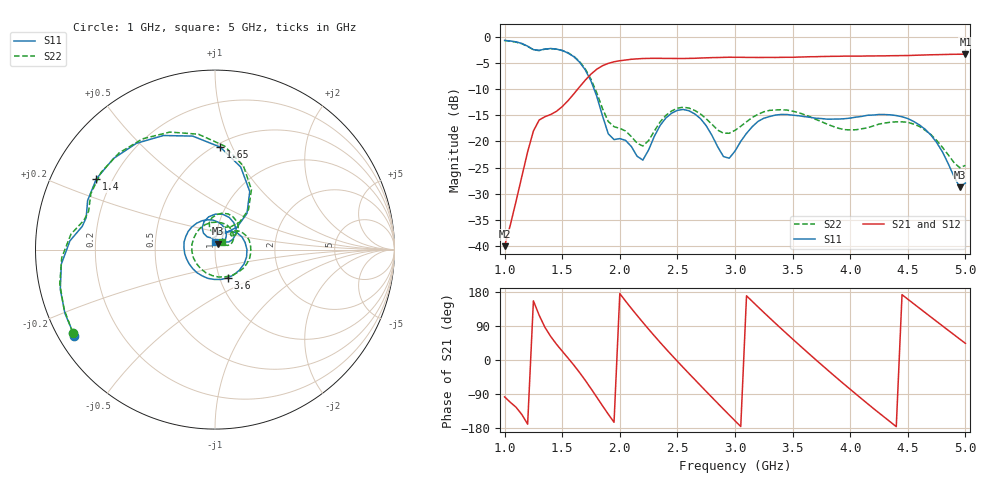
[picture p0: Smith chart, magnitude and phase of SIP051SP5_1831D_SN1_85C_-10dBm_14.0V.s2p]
# GHz  S  dB  R  50
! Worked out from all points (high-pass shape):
!   81 points, 1 GHz to 5 GHz, reference 50 ohm
!   highest |S21| = -3.36 dB at 5 GHz (marker M1); lowest = -40.0 dB at 1 GHz (marker M2)
!   |S21| within 3 dB of the highest: 1.793 GHz to end of sweep
!   lowest |S11| = -28.7 dB at 4.95 GHz (marker M3), VSWR 1.08, Z = 51.6 + j3.36 ohm
!   |S11| at or under -10 dB: 1.776 GHz to end of sweep
!   |S22| runs from -25.0 to -0.7 dB; largest |S21 - S12| = 0.0023
!   S11 on the Smith chart (normalised r, x): 1 GHz: 0.05, -0.28; 1.4 GHz: 0.14, +0.27; 1.65 GHz: 0.53, +0.90; 3.6 GHz: 1.09, -0.35; 5 GHz: 1.00, +0.08
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1  -0.73 -148.5  -40.01 -97.3  -39.77 -95.5  -0.74 -149.7
1.25  -2.49 170.1  -18.03 156.1  -18.01 156.1  -2.52 167.3
1.4  -2.27 149.2  -14.87 62.1  -14.87 62.2  -2.31 145.9
1.65  -4.86 87.1  -9.62 -32.8  -9.61 -32.7  -4.74 84.7
1.7  -6.34 72.7  -8.32 -53.6  -8.31 -53.5  -6.17 71.1
1.85  -15.15 45.5  -5.55 -120.9  -5.55 -120.9  -13.76 48.1
2  -19.47 78.3  -4.60 175.3  -4.59 175.3  -17.52 68.5
2.2  -23.57 104.6  -4.18 99.3  -4.19 99.4  -20.89 88.0
2.35  -16.97 120.3  -4.15 46.4  -4.14 46.5  -16.28 102.0
2.5  -14.08 89.5  -4.18 -3.5  -4.18 -3.5  -13.67 78.5
2.7  -15.65 44.6  -4.09 -67.2  -4.08 -67.2  -14.76 44.8
2.85  -21.05 28.9  -4.00 -114.2  -3.98 -114.2  -17.85 36.3
3  -21.85 59.8  -3.95 -160.4  -3.93 -160.5  -17.90 46.4
3.15  -17.19 47.0  -3.97 154.7  -3.97 154.6  -15.43 37.4
3.3  -15.26 12.9  -3.97 111.3  -3.98 111.2  -14.09 14.9
3.6  -15.27 -65.7  -3.88 28.0  -3.88 28.0  -14.89 -44.7
3.7  -15.58 -91.3  -3.84 1.0  -3.83 1.0  -15.80 -69.1
4.05  -15.38 -172.4  -3.73 -90.0  -3.72 -90.0  -17.78 -176.2
4.35  -14.94 124.9  -3.65 -163.8  -3.66 -163.8  -16.35 97.8
4.7  -18.78 57.1  -3.47 113.5  -3.46 113.6  -18.69 28.4
4.95  -28.74 62.9  -3.37 55.4  -3.37 55.4  -25.03 35.1
5  -27.95 87.2  -3.36 43.9  -3.36 43.8  -24.58 47.0
